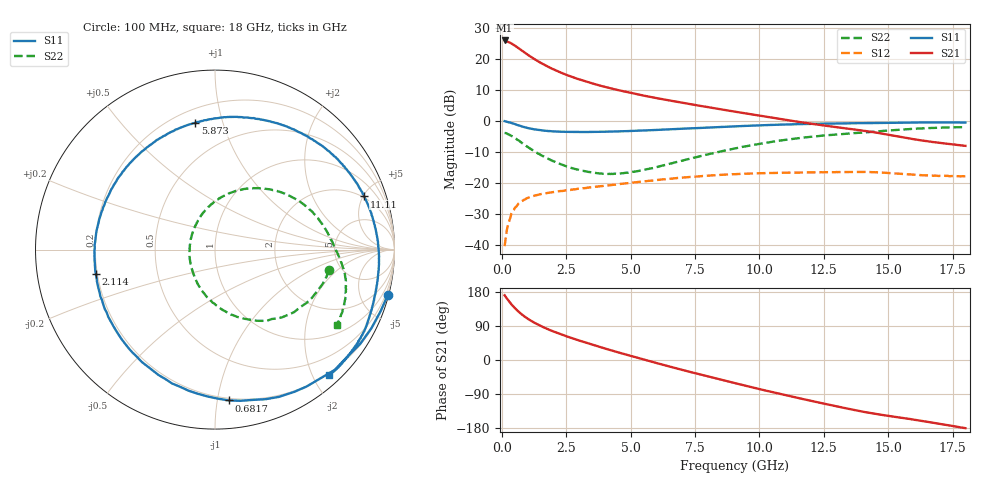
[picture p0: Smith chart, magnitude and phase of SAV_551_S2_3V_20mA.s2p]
! Data provided by Modelithics, Inc.  Tampa, Florida USA, June 2008
!Model SAV-551+
!VAR V_out= 3
!VAR I_out= 20
!VAR V_in= 0.3406
!VAR I_in= 0.8147
!BEGIN ACDATA
# GHZ S MA R 50
! Scattering Parameters
!% F n11x n11y n21x n21y n12x n12y n22x n22y
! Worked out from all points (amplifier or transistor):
!   401 points, 100 MHz to 18 GHz, reference 50 ohm
!   highest |S21| = 25.9 dB at 100 MHz (marker M1)
!   |S21| within 3 dB of that: start of sweep to 725.7 MHz
!   unconditionally stable (mu >= 1): 4.322 GHz to 10.34 GHz; 10.4741 GHz to 10.49175 GHz
!   at 3.054 GHz: K = 0.83, MSG = 17.5 dB, |S12| = -21.7 dB
!   at 9.05 GHz: K = 1.05, MAG = 8.6 dB, |S12| = -17.1 dB
!   at 18 GHz: K = 0.88, MSG = 4.9 dB, |S12| = -17.8 dB
!   lowest NFmin = 0.07 dB at 500 MHz
!   S11 on the Smith chart (normalised r, x): 100 MHz: 0.13, -7.80; 681.8 MHz: 0.18, -1.08; 2.114 GHz: 0.19, -0.10; 5.873 GHz: 0.28, +0.82; 11.11 GHz: 1.91, +5.08; 18 GHz: 0.17, -2.24
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0.1  0.9957 -14.6  19.72 170.8  0.00975 82.4  0.6433 -10.3
0.1895  0.9752 -26.7  18.96 162.1  0.01802 75.4  0.6295 -17.8
0.32375  0.9457 -45.1  18.05 150.4  0.02817 65.5  0.5892 -30.5
0.41325  0.9176 -56.3  17.16 143.0  0.03548 60.7  0.5616 -38.4
0.5475  0.8798 -71.3  15.76 133.6  0.04183 54.0  0.5182 -47.7
0.68175  0.8437 -84.8  14.4 125.2  0.0489 47.5  0.4743 -56.9
0.816  0.8085 -96.9  13.13 117.7  0.05297 42.0  0.4313 -64.6
0.95025  0.7834 -107.7  12 111.1  0.05733 38.4  0.3949 -71.7
1.2635  0.7348 -128.8  9.858 98.1  0.06317 30.9  0.325 -85.6
1.6215  0.7029 -147.7  8.1 86.0  0.06811 24.9  0.2695 -99.3
2.11375  0.6781 -168.4  6.44 72.2  0.07312 19.1  0.2155 -115.9
2.56125  0.6692 176.4  5.409 61.2  0.07753 15.2  0.1837 -130.1
3.09825  0.6647 160.4  4.521 49.2  0.0826 11.2  0.1592 -147.1
4.396  0.6793 128.7  3.221 22.5  0.09539 1.4  0.1424 169.5
5.87275  0.7148 98.8  2.391 -5.6  0.1111 -10.7  0.1761 126.5
6.0965  0.7231 94.8  2.299 -9.7  0.1137 -12.7  0.1859 121.2
7.439  0.7654 72.0  1.827 -33.7  0.1274 -25.6  0.2568 93.6
9.05  0.8198 47.8  1.412 -61.0  0.1399 -42.4  0.3626 66.7
11.1085  0.8815 19.6  1.03 -94.3  0.148 -65.5  0.5058 37.4
12.04825  0.9002 8.1  0.9005 -108.4  0.1498 -76.0  0.5607 25.7
15.0465  0.9368 -23.1  0.5979 -147.9  0.146 -106.6  0.7062 -5.7
18  0.9439 -47.9  0.3991 -179.9  0.1295 -131.5  0.7976 -31.8
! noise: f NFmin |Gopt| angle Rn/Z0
0.5  0.073  0.3928  32.95  0.065
0.7  0.104  0.3953  42.06  0.059
0.9  0.134  0.398  51.08  0.054
1  0.15  0.3995  55.57  0.051
1.9  0.287  0.4147  95.05  0.038
2.4  0.364  0.425  116.3  0.036
3  0.455  0.439  141.1  0.038
3.9  0.593  0.4636  177.1  0.054
5  0.761  0.4993  -141.2  0.09
6  0.914  0.5373  -105.2  0.14
